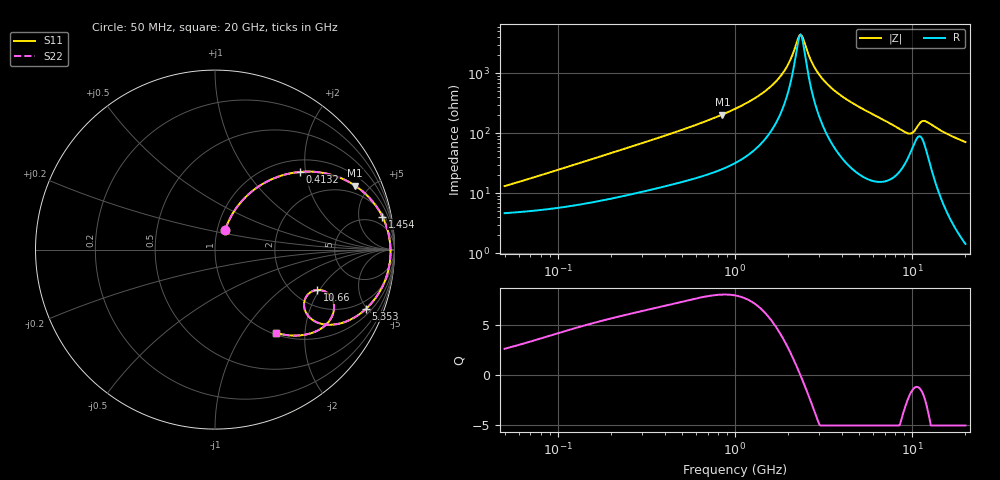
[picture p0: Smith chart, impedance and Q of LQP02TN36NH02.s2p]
!Murata Part Number: LQP02TN36NH02
!These Parameters are Measured in Series Mode Connection
!  o--[Z]--o
!Port1  Port2
!  o-------o
!Freq. Start=50[MHz] Stop=20[GHz], 401[Steps]
# Hz S RI R 50
!Freq.(Hz) S11(Real) S11(Imag) S21(Real) S21(Imag) S12(Real) S12(Imag) S22(Real) S22(Imag)
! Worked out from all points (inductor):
!   401 points, 50 MHz to 20 GHz, reference 50 ohm
!   read as one part in series: L = 38.6 nH near 59.85 MHz
!   highest Q = 8.04 at 848.1 MHz (marker M1), where L = 38.2 nH
!   self-resonance near 2.314 GHz
!   S11 on the Smith chart (normalised r, x): 50 MHz: 1.09, +0.25; 413.2 MHz: 1.27, +1.86; 1.454 GHz: 2.51, +9.59; 5.353 GHz: 1.37, -4.94; 10.66 GHz: 2.66, -1.91; 20 GHz: 1.03, -1.43
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5e7  0.0577 0.111  0.9423 -0.111  0.9423 -0.111  0.0577 0.111
1.364002e8  0.1403 0.2597  0.8597 -0.2597  0.8597 -0.2597  0.1403 0.2597
3.721004e8  0.4287 0.4267  0.5713 -0.4267  0.5713 -0.4267  0.4287 0.4267
4.132341e8  0.4729 0.4327  0.5271 -0.4327  0.5271 -0.4327  0.4729 0.4327
8.480927e8  0.781 0.356  0.219 -0.356  0.219 -0.356  0.781 0.356
1e9  0.8383 0.3107  0.1617 -0.3107  0.1617 -0.3107  0.8383 0.3107
1.454215e9  0.9327 0.1839  0.0673 -0.1839  0.0673 -0.1839  0.9327 0.1839
1.904239e9  0.9683 0.0816  0.0317 -0.0816  0.0317 -0.0816  0.9683 0.0816
2.05233e9  0.9735 0.0523  0.0265 -0.0523  0.0265 -0.0523  0.9735 0.0523
2.313601e9  0.9778 0.00494  0.0222 -0.00494  0.0222 -0.00494  0.9778 0.00494
2.419936e9  0.978 -0.013  0.022 0.013  0.022 0.013  0.978 -0.013
2.728004e9  0.9752 -0.061  0.0248 0.061  0.0248 0.061  0.9752 -0.061
3.029571e9  0.9683 -0.1034  0.0317 0.1034  0.0317 0.1034  0.9683 -0.1034
3.519108e9  0.9507 -0.1642  0.0493 0.1642  0.0493 0.1642  0.9507 -0.1642
5.352748e9  0.8424 -0.3289  0.1576 0.3289  0.1576 0.3289  0.8424 -0.3289
7.442007e9  0.6694 -0.4169  0.3306 0.4169  0.3306 0.4169  0.6694 -0.4169
9.457416e9  0.5 -0.3342  0.5 0.3342  0.5 0.3342  0.5 -0.3342
1.066139e10  0.5704 -0.2243  0.4296 0.2243  0.4296 0.2243  0.5704 -0.2243
1.149051e10  0.6533 -0.2742  0.3467 0.2742  0.3467 0.2742  0.6533 -0.2742
1.238412e10  0.6558 -0.3627  0.3442 0.3627  0.3442 0.3627  0.6558 -0.3627
1.482269e10  0.5341 -0.4662  0.4659 0.4662  0.4659 0.4662  0.5341 -0.4662
2e10  0.3421 -0.4645  0.6579 0.4645  0.6579 0.4645  0.3421 -0.4645
